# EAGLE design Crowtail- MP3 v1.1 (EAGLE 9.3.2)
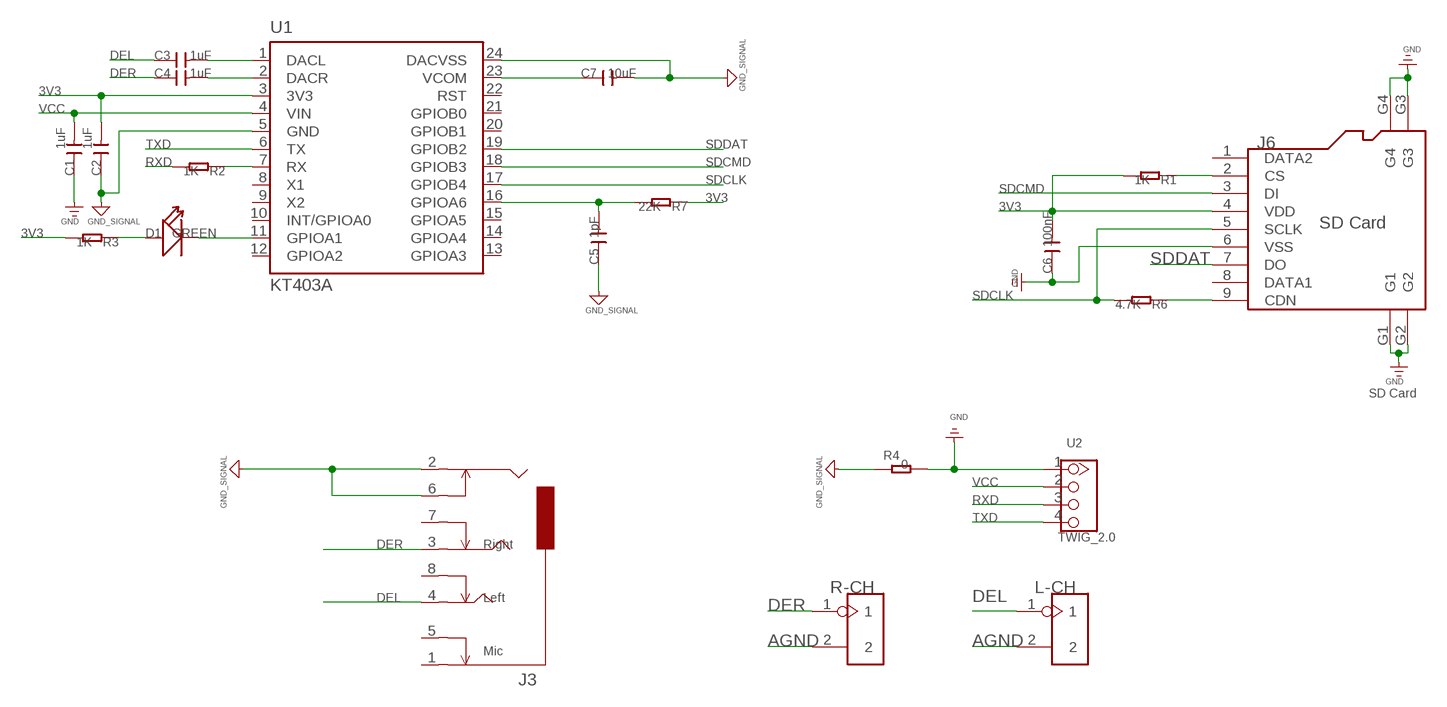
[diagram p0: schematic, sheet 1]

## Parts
C1  1uF  C-0603  [C0603]
C2  1uF  C-0603  [C0603]
C3  1uF  C-0603  [C0603]
C4  1uF  C-0603  [C0603]
C5  1pF  C-0603  [C0603]
C6  100nF  C-0603  [C0603]
C7  10uF  C-0603  [C0603]
D1  GREEN  LED'0805'  [LED-0805]
J3  AUDIO-8P-SMD'PJ-3536-L6S'  [8P-3.5-SMD]
J6  SD Card  HOLDER-MICROSD-9P  [9P-SMD-W/-RING]
L-CH  HEADER-2P-65/35MIL  [2P-2.54-65/35MIL]
R1  1K  R-0603  [R0603]
R2  1K  R-0603  [R0603]
R3  1K  R-0603  [R0603]
R4  0  R-0603  [R0603]
R6  4.7K  R-0603  [R0603]
R7  22K  R-0603  [R0603]
R-CH  HEADER-2P-65/35MIL  [2P-2.54-65/35MIL]
U1  KT403A  [SSOP24]
U2  TWIG_2.0  [2.0_1X4]

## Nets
3V3: C2.2 C6.2 J6.4(VDD) R1.2 R3.2 R7.1 U1.3(3V3)
AGND: C2.1 C5.1 C7.2 J3.2 J3.6 L-CH.2 R4.1 R-CH.2 U1.5(GND) U1.24(DACVSS) ; supply symbol labelled GND_SIGNAL
DEL: C3.1 J3.4 L-CH.1
DER: C4.1 J3.3 R-CH.1
GND: C1.1 C6.1 J6.6(VSS) J6.G1 J6.G2 J6.G3 J6.G4 R4.2 U2.1
N$1: C3.2 U1.1(DACL)
N$2: C4.2 U1.2(DACR)
N$3: D1.- U1.11(GPIOA1)
N$4: D1.+ R3.1
N$5: R2.1 U1.7(RX)
N$6: C7.1 U1.23(VCOM)
N$7: J6.2(CS) R1.1
N$8: J6.9(CDN) R6.1
N$10: C5.2 R7.2 U1.16(GPIOA6)
RXD: R2.2 U2.3
SDCLK: J6.5(SCLK) R6.2 U1.17(GPIOB4)
SDCMD: J6.3(DI) U1.18(GPIOB3)
SDDAT: J6.7(DO) U1.19(GPIOB2)
TXD: U1.6(TX) U2.4
VCC: C1.2 U1.4(VIN) U2.2
Unconnected: J3.1 J3.5 J3.7 J3.8 J6.1(DATA2) J6.8(DATA1) U1.8(X1) U1.9(X2) U1.10(INT/GPIOA0) U1.12(GPIOA2) U1.13(GPIOA3) U1.14(GPIOA4) U1.15(GPIOA5) U1.20(GPIOB1)

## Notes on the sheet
- SD Card
- Right
- Left
- Mic

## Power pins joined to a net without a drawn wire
GPIOB0: U1.21(GPIOB0)
RST: U1.22(RST)

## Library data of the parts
C1-C7 = Discrete:C*: Ceramic Capacitors
D1 = Discrete:LED*
J3 = Connector:AUDIO-8P-SMD
J6 = Connector:HOLDER-MICROSD-9P
L-CH R-CH = Connector:HEADER-2P
R1-R4 R6 R7 = Discrete:R*
U1 = KT403a :KT403A
U2 = CONNECTER:TWIG_2.0

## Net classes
1 power: width 0.61 mm, drill 0.406 mm, clearance 0.203 mm
2 gnd: width 0.305 mm, drill 0.559 mm, clearance 0.254 mm
3 usbvcc: width 0.508 mm, drill 0.61 mm, clearance 0.254 mm

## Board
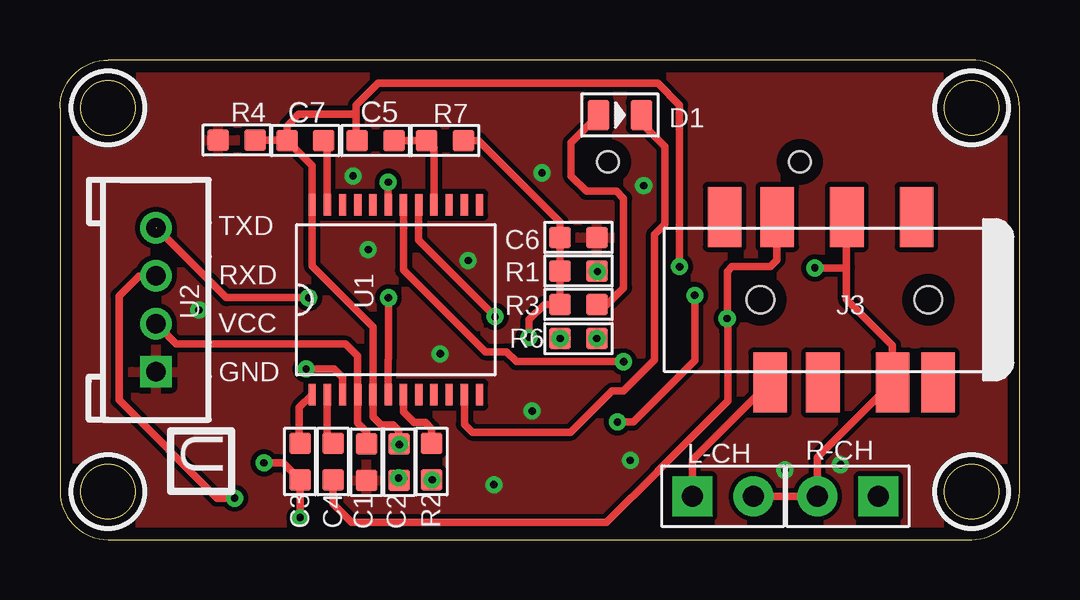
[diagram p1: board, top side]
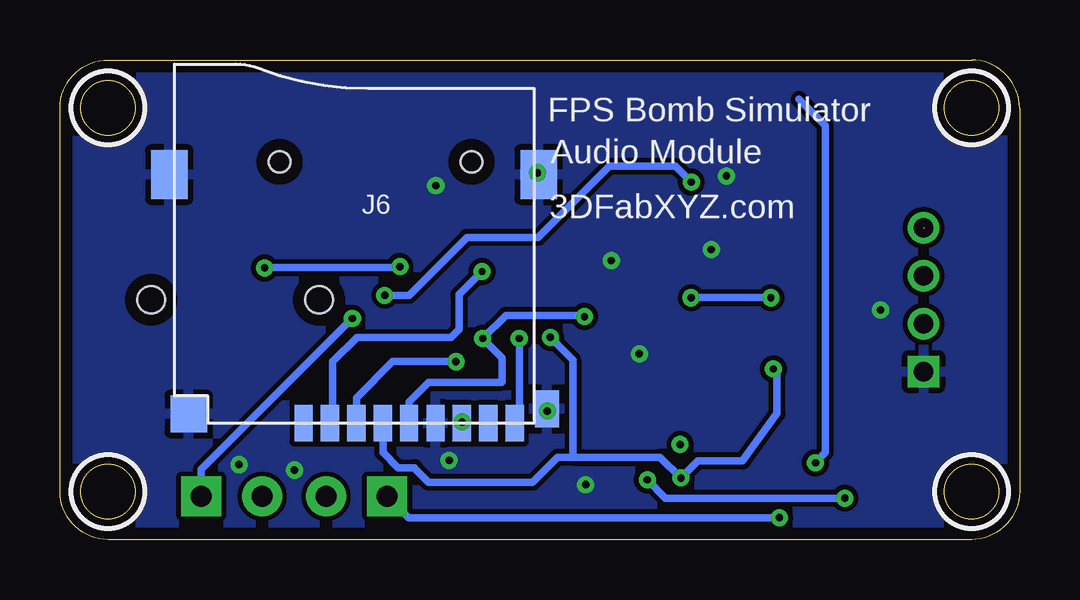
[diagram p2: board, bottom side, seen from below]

Size 40 x 20 mm. Coordinates in mm from the lower left corner, seen from the top.
Outline: 0,18 0,2 arc90 2,0 38,0 arc90 40,2 40,18 arc90 38,20 2,20 arc90 0,18
Outline: circle at 2,18 radius 1.14
Outline: circle at 2,2 radius 1.14
Outline: circle at 38,18 radius 1.14
Outline: circle at 38,2 radius 1.14
Copper layers (1*16): Top 0.035mm / dielectric 1.5mm / Bottom 0.035mm
Design rules "default": minimum track width 10mil, minimum drill 12mil, track to track 8mil, track to pad 8mil, pad to pad 8mil, via to via 8mil, smd to smd 0mil, copper to edge 20mil, drill to drill 8mil, minimum pad ring 10mil, minimum via ring 8mil, stop-mask expansion 2mil, vias tented up to drill 100mil, thermal gap 10mil
tRestrict: area 0.5,16.5 to 3.5,19.5; area 0.5,0.5 to 3.5,3.5; area 36.5,16.5 to 39.5,19.5; area 36.5,0.5 to 39.5,3.5
bRestrict: area 0.5,16.5 to 3.5,19.5; area 0.5,0.5 to 3.5,3.5; area 36.5,16.5 to 39.5,19.5; area 36.5,0.5 to 39.5,3.5

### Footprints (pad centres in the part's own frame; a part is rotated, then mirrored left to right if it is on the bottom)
C0603 = smd 0.889 x 0.889: 1 -0.762,0; 2 0.762,0
LED-0805 = smd 0.889 x 1.27: + -0.889,0; - 0.889,0
8P-3.5-SMD = smd 1.4 x 2.5: 1 2.8,-3.45; 2 5.7,-3.45; 3 8.6,-3.45; 4 8.9,3.45; 5 1.9,3.45; 6 3.8,3.45; 7 6.7,3.45; 8 10.8,-3.45 | hole 1.149: 2.3,0; 9.3,0
9P-SMD-W/-RING = smd 1.524 x 0.762: 1 0,4.4; 2 0,3.3; 3 0,2.2; 4 0,1.1; 5 0,0; 6 0,-1.1; 7 0,-2.2; 8 0,-3.3; 9 0,-4.4 | smd 1.524 x 1.016: G1 0.6,-5.746 | smd 2.032 x 1.524: G2 10.373,-5.4; G3 10.373,10 | smd 1.524 x 1.524: G4 0.392,9.181 | hole 0.889: 10.9,-2.6; 10.9,5.4
2P-2.54-65/35MIL = drill 0.889 pad 1.651 square: 1 0,1.27 | drill 0.889 pad 1.651: 2 0,-1.27
R0603 = smd 0.889 x 0.889: 1 -0.762,0; 2 0.762,0
SSOP24 = smd 0.305 x 0.91: 1 -3.493,-3.96; 2 -2.857,-3.96; 3 -2.223,-3.96; 4 -1.587,-3.96; 5 -0.953,-3.96; 6 -0.318,-3.96; 7 0.318,-3.96; 8 0.953,-3.96; 9 1.587,-3.96; 10 2.223,-3.96; 11 2.857,-3.96; 12 3.493,-3.96; 13 3.493,3.96; 14 2.857,3.96; 15 2.223,3.96; 16 1.587,3.96; 17 0.953,3.96; 18 0.318,3.96; 19 -0.318,3.96; 20 -0.953,3.96; 21 -1.587,3.96; 22 -2.223,3.96; 23 -2.857,3.96; 24 -3.493,3.96
2.0_1X4 = drill 0.8 pad 1.27 square: 1 -3,0 | drill 0.8 pad 1.27: 2 -1,0; 3 1,0; 4 3,0

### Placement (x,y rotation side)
C1  12.78,3.23 90 top
C2  14.14,3.23 270 top
C3  10.01,3.25 90 top
C4  11.38,3.25 90 top
C5  13.16,16.64 0 top
C6  21.62,12.6 180 top
C7  10.24,16.64 180 top
D1  23.34,17.7 0 top
J3  38.5,10 180 top
J6  25.45,4.85 90 bottom
L-CH  27.64,1.8 90 top
R1  21.62,11.2 180 top
R2  15.49,3.25 270 top
R3  21.62,9.8 180 top
R4  7.37,16.66 180 top
R6  21.62,8.38 0 top
R7  16.05,16.64 180 top
R-CH  32.84,1.8 270 top
U1  14,10 0 top
U2  4,10 90 top

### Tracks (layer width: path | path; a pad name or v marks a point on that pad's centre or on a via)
3V3  (via drill 0.3)
  Top 0.305: C2.2 14.14,2.54 v14.12,2.56 | C6.2 R1.2 R3.2 | C6.2 20.83,12.6 | R7.1 17.45,16.64 20.85,13.23 C6.2 | C6.2 20.88,12.57 | v19.56,8.43 19.56,9.17 20.19,9.8 R3.2 | 20.88,9.8 R3.2 | v10.26,7.11 11.43,7.11 11.78,6.76 11.78,6.2 11.78,6.19 U1.3
  Bottom 0.305: J6.4 26.54,4.83 26.54,3.63 25.9,3 25.25,3 | J6.4 | J6.4 26.56,4.85 | 25.25,3 25.22,3 | 18.59,3.43 18.62,3.45 18.62,7.49 v19.56,8.43 | 14.12,2.72 v14.12,2.56 | 18.59,3.43 19.25,3.43 20.3,2.39 24.64,2.39 25.25,3 | v10.26,7.11 10.1,6.96 10.1,5.26 11.55,3.28 13.41,3.28 v14.12,2.56 | 18.59,3.43 14.99,3.43 v14.12,2.56
AGND  (via drill 0.3)
  Top 0.305: C7.2 9.47,17.25 9.95,17.73 12.32,17.73 12.34,17.7 | 32.79,11.35 32.79,10.01 34.7,8.1 J3.6 31.57,3.42 R-CH.2 L-CH.2 | 32.79,11.35 32.79,13.34 32.8,13.34 J3.2 | v31.47,11.33 32.77,11.33 32.79,11.35 | R4.1 9.37,16.66 9.42,16.61 9.45,16.61 C7.2 | v14.15,3.96 14.17,3.94 14.15,3.91 v14.15,3.96 | v14.15,3.96 14.15,3.98 C2.1 | v25.83,11.38 25.83,18.11 24.92,19.02 13.26,19.02 | 13.26,19.02 13.25,19.02 | 12.34,17.7 12.34,18.11 13.26,19.02 | 12.34,17.7 12.34,16.59 | 12.34,16.59 12.42,16.51 | C5.1 12.34,16.59 | C7.2 10.51,15.6 U1.24 10.52,11.4 13.05,8.87 U1.5 13.05,5.11 13.39,4.78 13.89,4.78 14.12,4.55 14.12,3.99 v14.15,3.96
  Bottom 0.305: v31.47,11.33 31.45,11.35 25.86,11.35 v25.83,11.38
DEL  (via drill 0.3)
  Top 0.305: L-CH.1 26.36,3.33 29.57,6.53 29.58,6.53 J3.4 | v8.5,3.2 9.3,3.2 C3.1 v10.01,0.91
  Bottom 0.305: v8.5,3.2 8.5,3.23 8.1,3.63 8.1,17.27 9.2,18.36 | v10.01,0.91 25.48,0.91 L-CH.1
DER  (via drill 0.3)
  Top 0.305: J3.3 29.9,11.66 29.62,11.38 28.02,11.38 27.81,11.18 v27.81,9.22 27.84,8.69 27.84,5.79 24.92,2.87 24.92,2.85 22.78,0.71 12.17,0.71 11.38,1.5 C4.1
  Bottom 0.305: v27.81,9.22 34.11,2.92 R-CH.1
GND  (via drill 0.3)
  other vias: 20.09,15.29 18.08,2.29 17.02,11.63 12.85,12.09 5.79,9.58 23.77,3.3 19.68,5.36 24.33,14.76 15.85,7.75 30.23,2.9 32.54,3.12 12.22,15.16
  pour Top: 0,20.32 40.64,20.32 40.64,0 0,0
  pour Bottom: 0,20.32 40.64,20.32 40.64,0 0,0
N$1
  Top 0.305: C3.2 9.97,4.05 9.97,5.51 U1.1
N$2
  Top 0.305: U1.2 11.14,4.25 C4.2
N$3
  Top 0.305: 24.21,18.03 D1.- | 24.18,17.6 24.18,17.42 25.22,16.38 25.22,13.16 24.79,12.72 24.79,7.49 23.5,6.2 23.01,6.2 21.29,4.47 17.2,4.47 16.86,4.81 U1.11 | 24.18,17.6 24.18,17.63 | 24.21,17.68 D1.- | D1.- 24.26,17.7 24.21,17.65 24.21,17.63 24.18,17.6
N$4
  Top 0.305: D1.+ 21.31,16.56 21.31,15.16 21.95,14.53 23.19,14.53 23.5,14.22 23.5,10.49 22.81,9.8 R3.1
N$5
  Top 0.305: U1.7 14.32,5.32 14.76,4.88 15.24,4.88 15.49,4.62 15.49,4.04 15.47,4.01 R2.1
N$6
  Top 0.305: U1.23 11.14,16.51 11.02,16.64 11.02,16.56 10.99,16.54 C7.1
N$7  (via drill 0.3)
  Top 0.305: R1.1 v22.4,11.18
  Bottom 0.305: J6.2 28.63,4.97 28.63,7.42 27.61,8.43 23.7,8.43 23.37,8.76 23.37,10.21 v22.4,11.18
N$8  (via drill 0.3)
  Bottom 0.305: R6.1 20.85,5.05 J6.9
  other vias: 20.85,8.38
N$10
  Top 0.305: C5.2 R7.2 15.59,16.34 U1.16
RXD  (via drill 0.3)
  Top 0.305: U2.3 3.3,11 2.46,10.16 2.46,5.82 6.55,1.73 v7.29,1.73 | R2.2 15.49,2.28 v15.51,2.49
  Bottom 0.305: v7.29,1.73 14.76,1.73 v15.52,2.49 v15.51,2.49
SDCLK  (via drill 0.3)
  Top 0.305: U1.17 14.95,12.48 v18.14,9.3
  Bottom 0.305: J6.5 25.45,5.75 24.64,6.55 21.59,6.55 21.57,6.58 21.57,7.57 R6.2 21.41,9.35 18.19,9.35 v18.14,9.3
  other vias: 22.38,8.38
SDCMD  (via drill 0.3)
  Top 0.305: v23.5,7.42 19.02,7.42 18.62,7.82 17.73,7.82 14.32,11.23 U1.18
  Bottom 0.305: J6.3 27.65,5.91 26.14,7.42 v23.5,7.42
SDDAT  (via drill 0.3)
  Top 0.305: U1.19 13.68,13.87 13.69,13.87 v13.69,14.91 | v23.24,4.9 23.9,4.9 26.47,7.47 26.47,8.68 v26.46,10.19
  Bottom 0.305: 23.14,4.9 v23.24,4.9 23.24,4.88 23.27,4.85 J6.7 | 26.49,10.19 v26.46,10.19 25.45,10.19 23.04,12.6 20.07,12.6 17.09,15.57 14.35,15.57 v13.69,14.91
TXD  (via drill 0.3)  (1 unrouted)
  Top 0.305: U1.6 13.69,6.19 13.69,8.84 v13.69,10.08 | v10.36,10.08 6.93,10.08 4.01,13.01
  Bottom 0.305: v13.69,10.08 v10.36,10.08
VCC
  Top 0.305: U2.2 4.85,8.15 11.91,8.15 12.41,7.65 U1.4 12.41,4.86 12.78,4.5 C1.2 | C1.2 12.8,3.99 | C1.2 12.78,3.97 12.77,3.96 12.77,4.01

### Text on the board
tPlace: TXD | RXD | VCC | GND | U
bPlace: FPS Bomb Simulator | Audio Module | 3DFabXYZ.com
